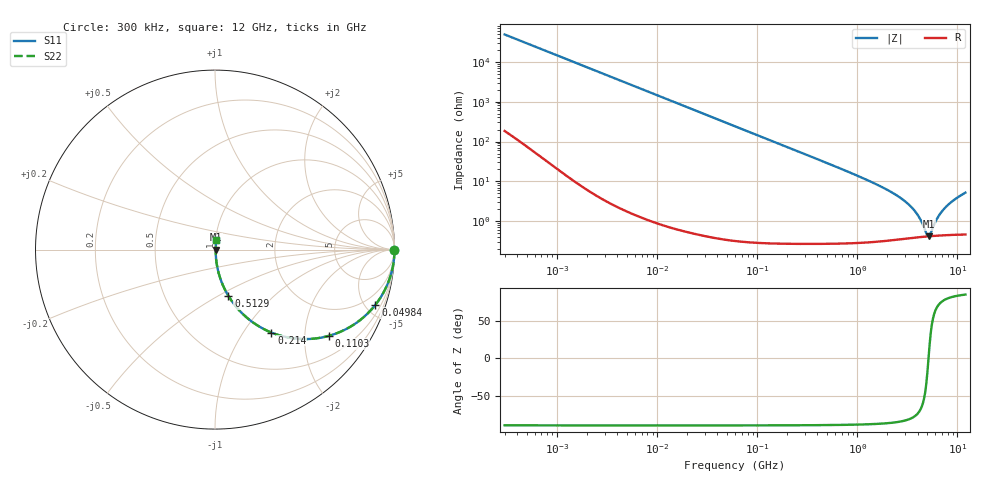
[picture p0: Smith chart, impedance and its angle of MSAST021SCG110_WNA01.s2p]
! MSAST021SCG110_WNA01  S-PARAMETER MODEL  ( Standard Model )
! Model Generated by TAIYO YUDEN Corporation (http://www.ty-top.com)
! Version 1.0
! TAIYO YUDEN Control No. 241126
! Copyright(c) 2024 TAIYO YUDEN CO.,LTD. All Rights Reserved.
! Product Description (link to TY-COMPAS)
! https://ds.yuden.co.jp/TYCOMPAS/or/detail?pn=MSAST021SCG110JWNA01&u=M
! Products Name : Multilayer Ceramic Capacitors
! Characteristics :
!  Capacitance : 11 [pF] , Rated Voltage : 25 [V] , TCC : CG / C0G
!  Case Size : 0.25 x 0.125 / 0.0098 x 0.0049 [mm/inch] , Thickness : 0.125 / 0.0049 [mm/inch]
!  (Conditions: Temperature = 25 [degC] , DC Bias Voltage = 0 [V])
! External Node Assignments :
!  1  o---| |---o  2
! GND o---------o GND
! Frequency Range : 0.3MHz  -  12000MHz  [ 401 STEP ]
# MHZ S RI R 50
! Freq[MHz].  S11 Real  S11 Imag  S21 Real  S21 Imag  S12 Real  S12 Imag  S22 Real  S22 Imag
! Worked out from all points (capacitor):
!   401 points, 300 kHz to 12 GHz, reference 50 ohm
!   read as one part in series: C = 11 pF near 316.3 kHz
!   lowest |Z| = 420 mohm at 5.141 GHz (marker M1)
!   series resonance near 5.14 GHz, so ESL is about 87 pH
!   S11 on the Smith chart (normalised r, x): 300 kHz: open; 49.84 MHz: 1.01, -5.82; 110.3 MHz: 1.01, -2.63; 214 MHz: 1.01, -1.35; 512.9 MHz: 1.01, -0.56; 12 GHz: 1.01, +0.10
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0.3  1 -0.00207  1.22e-05 0.00207  1.22e-05 0.00207  1 -0.00207
1.769972  0.9998 -0.0122  0.00016 0.0122  0.00016 0.0122  0.9998 -0.0122
10.44266  0.9948 -0.0717  0.00521 0.0717  0.00521 0.0717  0.9948 -0.0717
23.73947  0.9738 -0.1594  0.0262 0.1594  0.0262 0.1594  0.9738 -0.1594
49.84427  0.8941 -0.3072  0.1059 0.3072  0.1059 0.3072  0.8941 -0.3072
60  0.8535 -0.353  0.1465 0.353  0.1465 0.353  0.8535 -0.353
110.3493  0.6329 -0.4809  0.3671 0.4809  0.3671 0.4809  0.6329 -0.4809
213.9924  0.3147 -0.4624  0.6853 0.4624  0.6853 0.4624  0.3147 -0.4624
353.9943  0.1441 -0.3479  0.8559 0.3479  0.8559 0.3479  0.1441 -0.3479
512.9422  0.0747 -0.2581  0.9253 0.2581  0.9253 0.2581  0.0747 -0.2581
1166.079  0.0164 -0.1153  0.9836 0.1153  0.9836 0.1153  0.0164 -0.1153
2088.533  0.00653 -0.0568  0.9935 0.0568  0.9935 0.0568  0.00653 -0.0568
2870.14  0.00475 -0.034  0.9952 0.034  0.9952 0.034  0.00475 -0.034
3547.679  0.00425 -0.0208  0.9957 0.0208  0.9957 0.0208  0.00425 -0.0208
4050.141  0.00413 -0.0132  0.9959 0.0132  0.9959 0.0132  0.00413 -0.0132
4875.354  0.00414 -0.00289  0.9959 0.00289  0.9959 0.00289  0.00414 -0.00289
5140.631  0.00418 3.29e-06  0.9958 -3.29e-06  0.9958 -3.29e-06  0.00418 3.29e-06
5420.343  0.00423 0.00289  0.9958 -0.00289  0.9958 -0.00289  0.00423 0.00289
6354.153  0.00448 0.0116  0.9955 -0.0116  0.9955 -0.0116  0.00448 0.0116
7254.098  0.0048 0.0191  0.9952 -0.0191  0.9952 -0.0191  0.0048 0.0191
9207.246  0.00567 0.0334  0.9943 -0.0334  0.9943 -0.0334  0.00567 0.0334
12000  0.00731 0.0514  0.9927 -0.0514  0.9927 -0.0514  0.00731 0.0514
